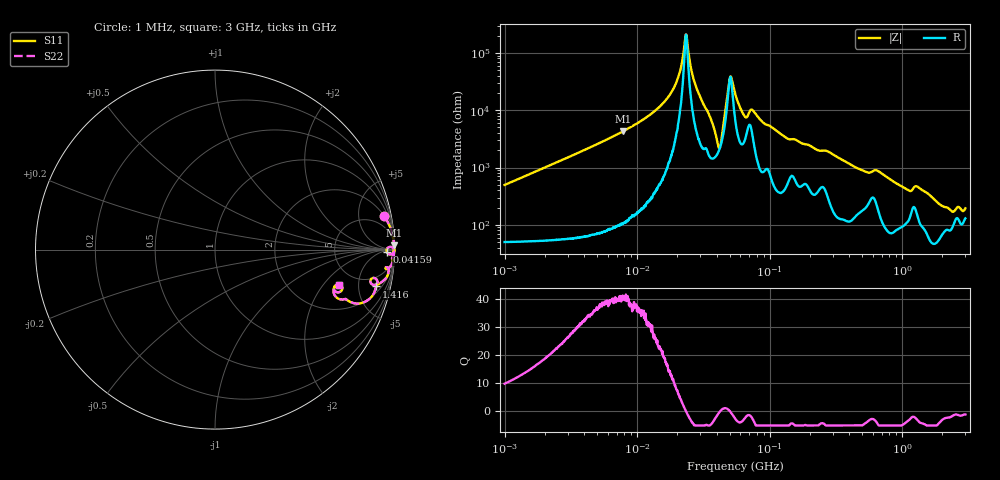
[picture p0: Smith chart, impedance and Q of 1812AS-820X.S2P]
!s-Parameter Generated by FASTRON Sdn. Bhd.
!FASTRON P/N : 1812AS-820X
!Keysight Technologies,E4991B,MY54100416,A.01.15
!Date created: Mon Oct 16 10:27:53 2023
!Version  : Rev00 Mon Oct 16 10:27:53 2023
!Data & Calibration Information:
!Freq	S11	S21	S12	S22
!PortZ  Port1:50+j0  Port2:50+j0
!When reading, reference impedance value at option line is always used.
! Remarks : This data is being provided solely for informational purposes.
# Hz S dB R 50
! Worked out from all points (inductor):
!   1601 points, 1 MHz to 3 GHz, reference 50 ohm
!   read as one part in series: L = 78.5 uH near 1.041 MHz
!   highest Q = 40.9 at 7.82 MHz (marker M1), where L = 87.1 uH
!   self-resonance near 23.39 MHz
!   S11 on the Smith chart (normalised r, x): 1 MHz: 2, +10; 41.59 MHz: 41, -15; 1.416 GHz: 2.85, -7.84; 3 GHz: 3.59, -2.89
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1000000  -0.34 11.1  -14.27 -73.1  -14.27 -73.1  -0.34 11.1
3804036  -0.03 3.0  -25.69 -85.2  -25.69 -85.2  -0.03 3.0
7819618  -0.01 1.3  -32.63 -87.2  -32.63 -87.2  -0.01 1.3
1.447069e7  -0.00 0.5  -40.82 -87.0  -40.82 -87.0  -0.00 0.5
1.953805e7  -0.00 0.2  -49.18 -83.2  -49.18 -83.2  -0.00 0.2
2.351201e7  -0.00 -0.0  -66.41 9.5  -66.41 9.5  -0.00 -0.0
2.732032e7  -0.01 -0.2  -49.23 78.7  -49.23 78.7  -0.01 -0.2
3.561766e7  -0.02 -0.7  -37.51 77.7  -37.51 77.7  -0.02 -0.7
4.159437e7  -0.37 -0.9  -27.03 19.2  -27.03 19.2  -0.37 -0.9
4.351043e7  -0.21 0.9  -30.87 -32.2  -30.87 -32.2  -0.21 0.9
5.005449e7  -0.02 0.0  -51.17 -6.8  -51.17 -6.8  -0.02 0.0
5.183886e7  -0.02 -0.1  -50.75 39.8  -50.75 39.8  -0.02 -0.1
5.477226e7  -0.02 -0.3  -45.95 68.3  -45.95 68.3  -0.02 -0.3
6.525633e7  -0.05 -0.7  -37.75 65.5  -37.75 65.5  -0.05 -0.7
7.395247e7  -0.03 -0.5  -40.15 67.4  -40.15 67.4  -0.03 -0.5
1.328058e8  -0.04 -1.7  -30.45 80.5  -30.45 80.5  -0.04 -1.7
2.083556e8  -0.07 -2.4  -27.31 78.8  -27.31 78.8  -0.07 -2.4
7.925923e8  -0.25 -8.6  -16.46 74.9  -16.46 74.9  -0.25 -8.6
1.108292e9  -0.79 -12.5  -12.96 61.1  -12.96 61.1  -0.79 -12.5
1.416254e9  -0.70 -12.9  -12.80 63.9  -12.80 63.9  -0.70 -12.9
1.970482e9  -1.69 -21.2  -8.47 52.0  -8.47 52.0  -1.69 -21.2
3e9  -2.90 -15.9  -8.68 32.2  -8.68 32.2  -2.90 -15.9
